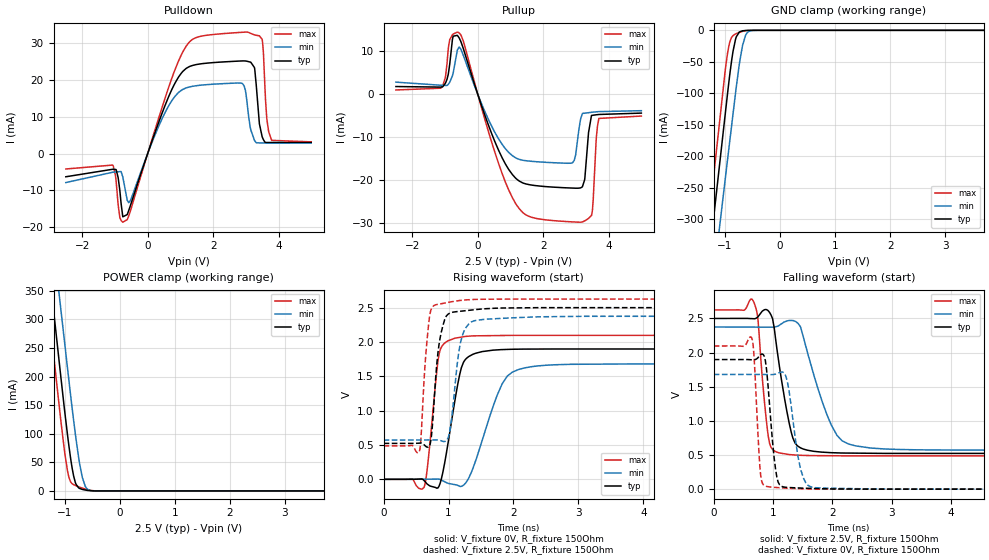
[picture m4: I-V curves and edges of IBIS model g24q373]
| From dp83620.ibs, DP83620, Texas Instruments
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|   Model g24q373
[Model]   g24q373
Model_type   I/O
Polarity   Non-Inverting
Vinl = 0.8
Vinh = 2.0
Vmeas = 1.25
Vref = 2.5
Cref = 15pF
Rref = 150
|   typ   min   max
|   (slow PVT)   (nom PVT)   (fast PVT)
C_comp   0.448p   0.445p   0.450p
|C_comp (ON state)   0.448p   0.445p   0.450p
|C_comp (OFF state)   0.441p   0.438p   0.444p
[Voltage Range]   2.5   2.375   2.625
[Temperature Range]   27   125   -40
[Pullup Reference]   2.5   2.375   2.625
[Pulldown Reference]   0   0   0
[Power Clamp Reference]   2.5   2.375   2.625
[GND Clamp Reference]   0   0   0
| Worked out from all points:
|   slope of the pulldown table from 0 to 0.375 V, typ, clamps not added: 39.9 ohm
|   slope of the pullup table from 0 to 0.375 V, typ, clamps not added: 46 ohm
|   GND clamp passes 1 mA (typ) near -0.68 V on its own axis
|   POWER clamp passes 1 mA (typ) near -0.59 V on its own axis
|   falling waveform, V_fixture 2.5V, R_fixture 150Ohm: 20-80 % time 227ps typ, 410ps min, 128ps max; typ from 2.5 V to 0.523 V
|   rising waveform, V_fixture 0V, R_fixture 150Ohm: 20-80 % time 203ps typ, 364ps min, 130ps max; typ from 0 V to 1.9 V
|   rising waveform, V_fixture 2.5V, R_fixture 150Ohm: 20-80 % time 118ps typ, 137ps min, 93ps max; typ from 0.523 V to 2.5 V
|   falling waveform, V_fixture 0V, R_fixture 150Ohm: 20-80 % time 115ps typ, 169ps min, 74.9ps max; typ from 1.9 V to 0 V
[Pulldown]
|   Voltage   I(typ)   I(min)   I(max)
-2.5V     -6.301mA   -7.87mA    -4.193mA
-1.067V   -4.261mA   -5.073mA   -3.123mA
-850mV    -10.03mA   -4.9mA     -17.38mA
-625mV    -16.56mA   -12.65mA   -17.93mA
957.5mV   20.95mA    16.67mA    25.42mA
1.895V    24.59mA    18.74mA    32.18mA
2.9V      25.12mA    18.92mA    32.89mA
3.147V    24.76mA    6.409mA    32.57mA
3.268V    22.92mA    3.458mA    32.16mA
3.41V     8.064mA    2.886mA    31.93mA
3.785V    2.989mA    2.887mA    3.573mA
4.992V    2.997mA    2.896mA    3.167mA
[GND Clamp]
|   Voltage   I(typ)   I(min)   I(max)
-2.5V     -1.339A    -1.384A    -1.315A
-1.66V    -661.3mA   -738.1mA   -610.7mA
-1.278V   -357.2mA   -448.8mA   -294.4mA
-1.21V    -303.9mA   -398.2mA   -238.9mA
-1.165V   -268.5mA   -364.6mA   -202mA
-992.5mV  -133.4mA   -236.7mA   -63.79mA
-940mV    -92.71mA   -198.1mA   -31.44mA
-850mV    -33.15mA   -132.4mA   -8.308mA
-730mV    -2.402mA   -50.04mA   -3.042mA
-625mV    -273.8uA   -8.504mA   -672.2uA
-497.5mV  -14.45uA   -281.2uA   -27.02uA
4.992V    0A         0A         0A
[Pullup]
|   Voltage   I(typ)   I(min)   I(max)
-2.5V     1.836mA    2.857mA    1.034mA
-1.127V   1.702mA    2.137mA    1.448mA
-857.5mV  7.029mA    2.836mA    12.75mA
-752.5mV  13.55mA    4.976mA    14.05mA
-572.5mV  13.18mA    11.02mA    14.33mA
950mV     -17.53mA   -13.54mA   -22.34mA
2.105V    -21.46mA   -15.81mA   -29.2mA
2.9V      -21.79mA   -15.83mA   -29.65mA
3.192V    -21.49mA   -4.43mA    -29.66mA
3.47V     -4.893mA   -4.159mA   -28.16mA
3.695V    -4.663mA   -3.998mA   -5.585mA
4.992V    -4.342mA   -3.781mA   -5.028mA
[POWER Clamp]
|   Voltage   I(typ)   I(min)   I(max)
-2.5V     1.468A     1.541A     1.422A
-1.165V   285.5mA    400.7mA    208.4mA
-1.157V   278.9mA    394.3mA    201.6mA
-1.075V   206.1mA    324.2mA    129.3mA
-992.5mV  135.3mA    254mA      63.99mA
-932.5mV  87.45mA    203mA      28.56mA
-835mV    26.06mA    123.1mA    10.98mA
-790mV    11.35mA    89.4mA     9.001mA
-722.5mV  4.146mA    45.6mA     6.498mA
-625mV    1.561mA    8.387mA    3.375mA
-490mV    160.1uA    282.6uA    541.7uA
4.992V    0A         0A         0A
[Ramp]
R_load = 150
|   typ   min   max
dV/dt_r   1.13883/2.03477e-10   1.00813/3.64153e-10   1.25786/1.29663e-10
dV/dt_f   1.18609/2.27326e-10   1.0822/4.10143e-10   1.28243/1.28436e-10
[Falling Waveform]
V_fixture = 2.5V
V_fixture_min = 2.375V
V_fixture_max = 2.625V
R_fixture = 150Ohm
C_fixture = 0F
|   Time   V(typ)   V(min)   V(max)
0s        2.5V       2.375V     2.625V
663.1ps   2.497V     2.373V     2.761V
742.6ps   2.522V     2.373V     2.516V
839.3ps   2.619V     2.373V     1.426V
940.9ps   2.589V     2.372V     672.8mV
1.267ns   991.2mV    2.469V     507.4mV
1.464ns   604.7mV    2.376V     496.3mV
2.08ns    531.6mV    786.8mV    488.8mV
2.641ns   525.7mV    603.1mV    487.9mV
19.9ns    523.2mV    571.3mV    487.6mV
[Rising Waveform]
V_fixture = 0V
V_fixture_min = 0V
V_fixture_max = 0V
R_fixture = 150Ohm
C_fixture = 0F
|   Time   V(typ)   V(min)   V(max)
0s        567.5pV    22.84nV    158pV
624.1ps   -18.33mV   2.409mV    -115.5mV
676.7ps   -72.62mV   2.613mV    193.8mV
835.8ps   -125.9mV   3.227mV    1.712V
919.7ps   138.5mV    -25.24mV   1.965V
1.17ns    1.52V      -100.2mV   2.067V
1.267ns   1.753V     -49.32mV   2.082V
1.826ns   1.889V     1.391V     2.094V
2.388ns   1.897V     1.653V     2.096V
19.9ns    1.898V     1.68V      2.096V
[Rising Waveform]
V_fixture = 2.5V
V_fixture_min = 2.375V
V_fixture_max = 2.625V
R_fixture = 150Ohm
C_fixture = 0F
|   Time   V(typ)   V(min)   V(max)
0s        523.2mV    571.3mV    487.6mV
547.4ps   526.4mV    572.7mV    399.1mV
704.3ps   482.7mV    573.1mV    2.35V
835.8ps   1.838V     572.4mV    2.548V
889.2ps   2.147V     560.3mV    2.558V
1.019ns   2.42V      695.4mV    2.581V
1.174ns   2.447V     1.942V     2.604V
1.383ns   2.468V     2.306V     2.619V
2.388ns   2.5V       2.366V     2.625V
19.9ns    2.5V       2.375V     2.625V
[Falling Waveform]
|Gnd
V_fixture = 0V
V_fixture_min = 0V
V_fixture_max = 0V
R_fixture = 150Ohm
C_fixture = 0F
|   Time   V(typ)   V(min)   V(max)
0s        1.898V     1.68V      2.096V
637.6ps   1.895V     1.68V      2.218V
792.7ps   1.971V     1.68V      191.4mV
869.9ps   1.884V     1.679V     45.96mV
940.9ps   1.238V     1.678V     33.1mV
1.086ns   103.2mV    1.699V     22.75mV
1.239ns   25.79mV    1.585V     14.23mV
1.464ns   16.35mV    296mV      6.494mV
1.691ns   9.976mV    23.86mV    2.57mV
19.9ns    4.14uV     -4.768uV   -7.42uV
